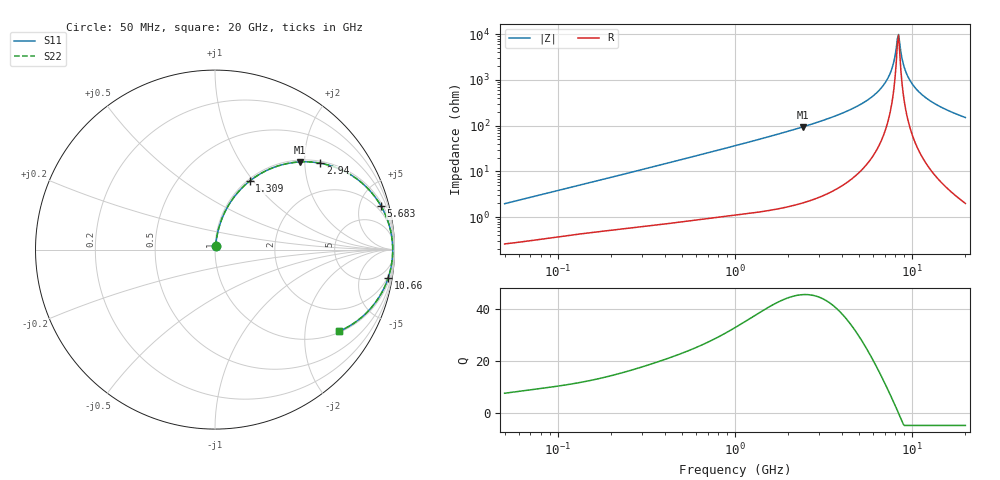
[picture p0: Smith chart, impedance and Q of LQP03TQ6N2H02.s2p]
!Murata Part Number: LQP03TQ6N2H02
!These Parameters are Measured in Series Mode Connection
!  o--[Z]--o
!Port1  Port2
!  o-------o
!Freq. Start=50[MHz] Stop=20[GHz], 401[Steps]
# Hz S RI R 50
!Freq.(Hz) S11(Real) S11(Imag) S21(Real) S21(Imag) S12(Real) S12(Imag) S22(Real) S22(Imag)
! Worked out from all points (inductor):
!   401 points, 50 MHz to 20 GHz, reference 50 ohm
!   read as one part in series: L = 6.19 nH near 51.52 MHz
!   highest Q = 45.8 at 2.42 GHz (marker M1), where L = 6.19 nH
!   self-resonance near 8.265 GHz
!   S11 on the Smith chart (normalised r, x): 50 MHz: 1.01, +0.04; 1.309 GHz: 1.03, +0.96; 2.94 GHz: 1.05, +2.39; 5.683 GHz: 1.32, +7.52; 10.66 GHz: 2, -12; 20 GHz: 1.04, -3.01
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5e7  0.00299 0.0195  0.997 -0.0195  0.997 -0.0195  0.00299 0.0195
1.364002e8  0.00695 0.0509  0.9931 -0.0509  0.9931 -0.0509  0.00695 0.0509
3.721004e8  0.0247 0.132  0.9753 -0.132  0.9753 -0.132  0.0247 0.132
1e9  0.1245 0.3153  0.8755 -0.3153  0.8755 -0.3153  0.1245 0.3153
1.309461e9  0.1939 0.3824  0.8061 -0.3824  0.8061 -0.3824  0.1939 0.3824
2.419936e9  0.4708 0.4883  0.5292 -0.4883  0.5292 -0.4883  0.4708 0.4883
2.728004e9  0.5414 0.4874  0.4586 -0.4874  0.4586 -0.4874  0.5414 0.4874
2.940159e9  0.5866 0.4814  0.4134 -0.4814  0.4134 -0.4814  0.5866 0.4814
4.275624e9  0.8031 0.3841  0.1969 -0.3841  0.1969 -0.3841  0.8031 0.3841
5.683258e9  0.925 0.2429  0.075 -0.2429  0.075 -0.2429  0.925 0.2429
6.701223e9  0.9683 0.1434  0.0317 -0.1434  0.0317 -0.1434  0.9683 0.1434
7.442007e9  0.984 0.0761  0.016 -0.0761  0.016 -0.0761  0.984 0.0761
7.784049e9  0.9878 0.0468  0.0122 -0.0468  0.0122 -0.0468  0.9878 0.0468
8.141811e9  0.9899 0.0172  0.0101 -0.0172  0.0101 -0.0172  0.9899 0.0172
8.389408e9  0.9902 -0.00252  0.00978 0.00252  0.00978 0.00252  0.9902 -0.00252
8.516016e9  0.9901 -0.0124  0.00989 0.0124  0.00989 0.0124  0.9901 -0.0124
8.907419e9  0.9886 -0.042  0.0114 0.042  0.0114 0.042  0.9886 -0.042
9.316812e9  0.9853 -0.0714  0.0147 0.0714  0.0147 0.0714  0.9853 -0.0714
9.892087e9  0.9781 -0.1103  0.0219 0.1103  0.0219 0.1103  0.9781 -0.1103
1.066139e10  0.9648 -0.158  0.0352 0.158  0.0352 0.158  0.9648 -0.158
1.375312e10  0.8852 -0.306  0.1148 0.306  0.1148 0.306  0.8852 -0.306
2e10  0.6918 -0.4552  0.3082 0.4552  0.3082 0.4552  0.6918 -0.4552
